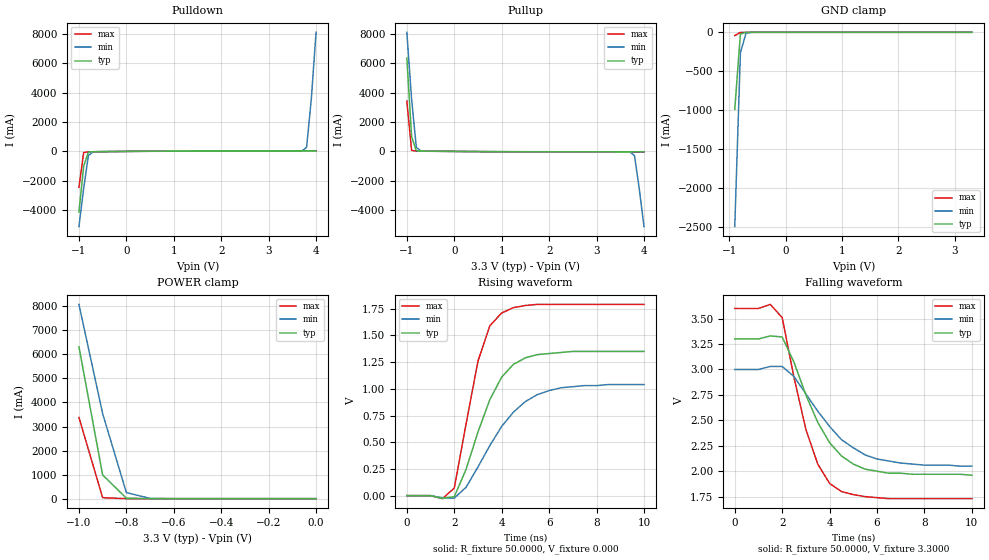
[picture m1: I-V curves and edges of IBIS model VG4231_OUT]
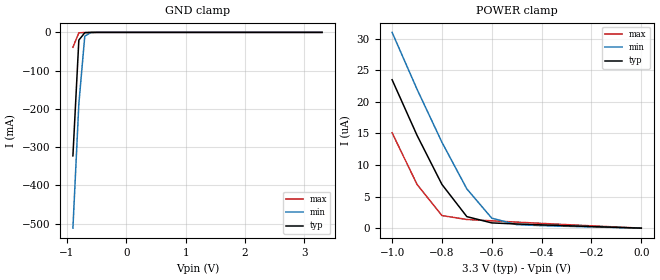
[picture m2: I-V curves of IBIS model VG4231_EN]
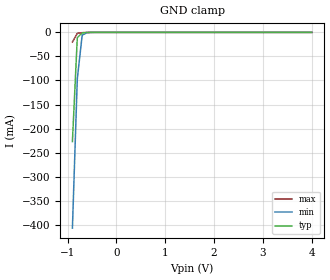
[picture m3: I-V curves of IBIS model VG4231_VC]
[IBIS ver]   2.1
[File name]   4231cacm.ibs
[File Rev]   0.1
[Date]   November 12, 2007
[Copyright]   EPSONTOYOCOM Corp.
|   Component VG-4231CAxxC
[Component]   VG-4231CAxxC
[Manufacturer]   EPSONTOYOCOM Corp.
[Package]
| variable   typ   min   max
R_pkg   0.20   0.13   0.28
L_pkg   5.16nH   4.56nH   5.76nH
C_pkg   1.23pF   1.03pF   1.53pF
[Pin]  signal_name   model_name   R_pin   L_pin   C_pin
1   VC   VG4231_VC
2   NC   NC
3   GND   GND
4   OUT   VG4231_OUT
5   OE   VG4231_EN
6   VDD   POWER
| Models and submodels in the file (3): VG4231_OUT (3-state), VG4231_EN (Input), VG4231_VC (Input)
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|   Model VG4231_OUT
[Model]   VG4231_OUT
Model_type   3-state
Polarity   Non-Inverting
Enable   Active-High
C_comp   2.2010pF   2.2010pF   2.2010pF
[Temperature Range]   27.0000   85.0000   -40.0000
[Voltage Range]   3.3000V   3.0000V   3.6000V
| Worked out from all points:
|   slope of the pulldown table from 0 to 0.495 V, typ, clamps not added: 42.7 ohm
|   slope of the pullup table from 0 to 0.495 V, typ, clamps not added: 46.2 ohm
|   GND clamp passes 1 mA (typ) near -0.70 V on its own axis
|   POWER clamp passes 1 mA (typ) near -0.70 V on its own axis
|   rising waveform, R_fixture 50.0000, V_fixture 0.000: 20-80 % time 1.4ns typ, 1.91ns min, 1.02ns max; typ from 0 V to 1.35 V
|   falling waveform, R_fixture 50.0000, V_fixture 3.3000: 20-80 % time 1.64ns typ, 2.08ns min, 1.21ns max; typ from 3.3 V to 1.96 V
[Pulldown]
| voltage   I(typ)   I(min)   I(max)
-1V       -4.11A     -5.11A     -2.44A
-900mV    -1.01A     -2.51A     -75.4mA
-800mV    -43.6mA    -277mA     -30.8mA
-700mV    -19.9mA    -25mA      -26.6mA
3.6V      27.8mA     20.4mA     39.8mA
3.7V      27.9mA     30.4mA     39.9mA
3.8V      27.9mA     274mA      39.9mA
3.9V      28mA       3.56A      39.9mA
4V        28.7mA     8.1A       40mA
[Pullup]
| voltage   I(typ)   I(min)   I(max)
-1V       6.35A      8.1A       3.42A
-900mV    1.01A      3.56A      71.5mA
-800mV    42.3mA     271mA      28.1mA
-700mV    19mA       25.3mA     24.1mA
-600mV    15.7mA     13.2mA     20.6mA
3.7V      -30.5mA    -33.8mA    -41.8mA
3.8V      -30.6mA    -284mA     -42mA
3.9V      -30.8mA    -2.52A     -42.1mA
4V        -31.7mA    -5.11A     -42.2mA
[GND_clamp]
| voltage   I(typ)   I(min)   I(max)
-900mV    -988mA     -2.49A     -42.8mA
-800mV    -22.3mA    -261mA     -1.3mA
-700mV    -968uA     -10.8mA    -315uA
-500mV    -14.7uA    -62uA      -1.68uA
3.3V      74.5pA     1.55uA     62.4pA
[POWER_clamp]
| voltage   I(typ)   I(min)   I(max)
-1V       6.32A      8.08A      3.38A
-900mV    985mA      3.54A      40.6mA
-800mV    21.5mA     254mA      540uA
-700mV    770uA      10.7mA     43.6uA
-600mV    84.6uA     712uA      4.3uA
-500mV    10.8uA     95.8uA     259nA
-400mV    1.01uA     13.7uA     7.7nA
-300mV    59.3nA     1.55uA     241pA
-200mV    2.49nA     124nA      92.5pA
-100mV    153pA      7.18nA     84.8pA
0V        74.5pA     170pA      79.2pA
[Ramp]
| variable   typ   min   max
dV/dt_r   0.81/1.40n   0.624/1.86n   1.08/0.95n
dV/dt_f   0.80/1.62n   0.578/2.04n   1.12/1.18n
R_load = 50.0000
[Rising Waveform]
R_fixture = 50.0000
V_fixture = 0.000
V_fixture_min = 0.000
V_fixture_max = 0.000
| time   V(typ)   V(min)   V(max)
0s        2.47nV     15.3nV     2.09nV
1.5ns     -25.3mV    -20.8mV    -28.3mV
2ns       -10mV      -23.1mV    70.9mV
2.5ns     248mV      79.1mV     674mV
3ns       596mV      269mV      1.26V
3.5ns     899mV      469mV      1.59V
4ns       1.11V      648mV      1.71V
5ns       1.29V      881mV      1.78V
6ns       1.33V      983mV      1.79V
10ns      1.35V      1.04V      1.79V
[Falling Waveform]
R_fixture = 50.0000
V_fixture = 3.3000
V_fixture_min = 3.0000
V_fixture_max = 3.6000
| time   V(typ)   V(min)   V(max)
0s        3.3V       3V         3.6V
1.5ns     3.33V      3.03V      3.64V
2ns       3.32V      3.03V      3.51V
2.5ns     3.07V      2.93V      2.92V
3ns       2.75V      2.76V      2.41V
3.5ns     2.48V      2.59V      2.07V
4ns       2.28V      2.44V      1.88V
5ns       2.07V      2.23V      1.77V
6ns       2V         2.12V      1.74V
10ns      1.96V      2.05V      1.73V
|   Model VG4231_EN
[Model]   VG4231_EN
Model_type   Input
Vinl =   0.6600V
Vinh =   2.6400V
C_comp   1.4070pF   1.4070pF   1.4070pF
[Temperature Range]   27.0000   85.0000   -40.0000
[Voltage Range]   3.3000V   3.0000V   3.6000V
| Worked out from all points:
|   GND clamp passes 1 mA (typ) near -0.70 V on its own axis
[GND_clamp]
| voltage   I(typ)   I(min)   I(max)
-900mV    -323mA     -512mA     -39mA
-800mV    -20.3mA    -187mA     -1.24mA
-700mV    -916uA     -9.88mA    -313uA
-600mV    -139uA     -599uA     -39.6uA
-500mV    -16.2uA    -62uA      -3.84uA
3.3V      18.4pA     290nA      -498nA
[POWER_clamp]
| voltage   I(typ)   I(min)   I(max)
-1V       23.5uA     31uA       15.1uA
-900mV    14.7uA     22uA       6.93uA
-800mV    6.92uA     13.6uA     1.99uA
-700mV    1.82uA     6.21uA     1.37uA
-600mV    828nA      1.58uA     1.16uA
-500mV    659nA      555nA      954nA
-400mV    518nA      396nA      753nA
-300mV    382nA      290nA      557nA
-200mV    250nA      189nA      366nA
-100mV    123nA      92.7nA     180nA
0V        18.4pA     119pA      18pA
|   Model VG4231_VC
[Model]   VG4231_VC
Model_type   Input
Vinl =   0.800V
Vinh =   2.000V
C_comp   1.4070pF   1.4070pF   1.4070pF
[Temperature Range]   27.0000   85.0000   -40.0000
[Voltage Range]   3.3000V   3.0000V   3.6000V
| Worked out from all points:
|   GND clamp passes 1 mA (typ) near -0.67 V on its own axis
[GND_clamp]
| voltage   I(typ)   I(min)   I(max)
-900mV    -227mA     -407mA     -20.1mA
-800mV    -11mA      -96.7mA    -2.11mA
-700mV    -1.25mA    -5.64mA    -622uA
-600mV    -265uA     -674uA     -75.4uA
-500mV    -29.8uA    -103uA     -3.49uA
4V        12.3pA     250pA      8pA
